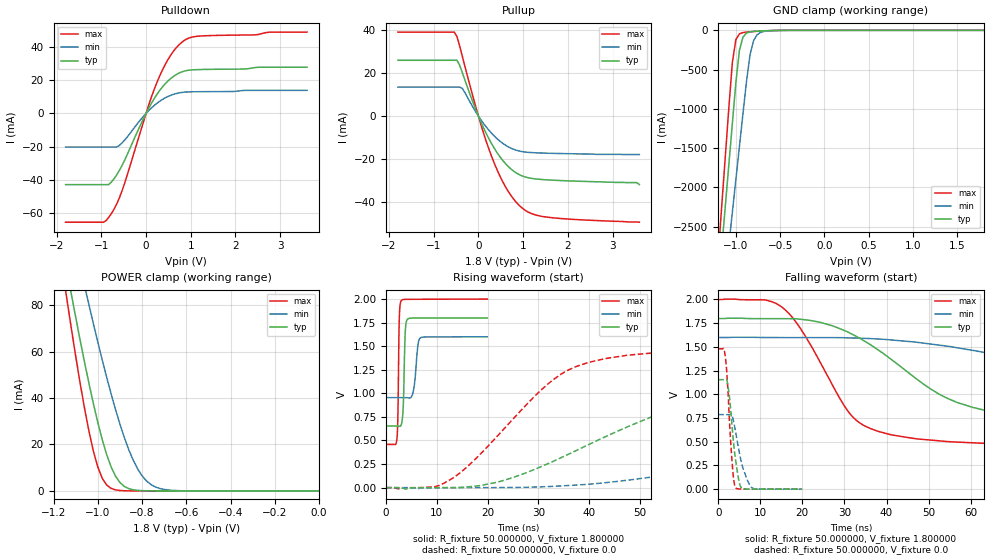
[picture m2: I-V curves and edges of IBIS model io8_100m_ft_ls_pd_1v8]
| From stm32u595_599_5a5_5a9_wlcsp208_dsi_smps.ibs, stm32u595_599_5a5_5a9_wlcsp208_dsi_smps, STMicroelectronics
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|   Model io8_100m_ft_ls_pd_1v8
[Model]  io8_100m_ft_ls_pd_1v8
Model_type I/O
Polarity   Non-Inverting
Enable   Active-Low
Vinl =   0.540000V
Vinh =   1.260000V
Vmeas =  0.900000V
Cref =   50.000000pF
Rref =   100.000000M
Vref =   0.0V
C_comp   3.148300pF   3.147400pF   3.196500pF
[Temperature Range]   25.000000   0.140000k   -40.000000
[Pullup Reference]   1.800000V   1.600000V   2.000000V
[Pulldown Reference]   0.0V   0.0V   0.0V
[POWER Clamp Reference]   1.800000V   1.600000V   2.000000V
[GND Clamp Reference]   0.0V   0.0V   0.0V
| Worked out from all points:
|   slope of the pulldown table from 0 to 0.27 V, typ, clamps not added: 21.7 ohm
|   slope of the pullup table from 0 to 0.27 V, typ, clamps not added: 22.6 ohm
|   GND clamp passes 1 mA (typ) near -0.51 V on its own axis
|   POWER clamp passes 1 mA (typ) near -0.86 V on its own axis
|   rising waveform, R_fixture 50.000000, V_fixture 1.800000: 20-80 % time 318ps typ, 631ps min, 230ps max; typ from 0.654 V to 1.8 V
|   rising waveform, R_fixture 50.000000, V_fixture 0.0: 20-80 % time 31.3ns typ, 66.8ns min, 16.5ns max; typ from 0 V to 1.15 V
|   falling waveform, R_fixture 50.000000, V_fixture 1.800000: 20-80 % time 24.6ns typ, 55.5ns min, 12.3ns max; typ from 1.8 V to 0.654 V
|   falling waveform, R_fixture 50.000000, V_fixture 0.0: 20-80 % time 1.6ns typ, 2.38ns min, 1.17ns max; typ from 1.15 V to 0 V
[Pulldown]
|Voltage   I(typ)   I(min)   I(max)
-1.8V     -42.74mA   -20.21mA   -65.25mA
-960mV    -42.74mA   -20.21mA   -65.25mA
-780mV    -41.3mA    -20.21mA   -60.25mA
-660mV    -37mA      -20.2mA    -54.5mA
-540mV    -31.39mA   -17.82mA   -46.65mA
0V        0A         0A         0A
240mV     11.28mA    6.002mA    18.38mA
480mV     19.17mA    10.02mA    31.83mA
780mV     24.67mA    12.5mA     42.21mA
960mV     25.9mA     12.9mA     45.21mA
1.14V     26.24mA    12.99mA    46.23mA
3.6V      27.67mA    13.81mA    48.75mA
[Pullup]
|Voltage   I(typ)   I(min)   I(max)
-1.8V     26.06mA    13.5mA     39.23mA
-540mV    26.06mA    13.5mA     39.23mA
-480mV    26.06mA    13.5mA     37.19mA
-360mV    20.34mA    12.93mA    27.94mA
0V        0A         0A         0A
300mV     -13.1mA    -8.158mA   -19.11mA
480mV     -18.98mA   -11.71mA   -27.97mA
660mV     -23.42mA   -14.29mA   -34.95mA
1.02V     -28.29mA   -16.75mA   -43.65mA
1.26V     -29.33mA   -17.15mA   -46.11mA
1.62V     -29.92mA   -17.41mA   -47.45mA
3.6V      -32mA      -18mA      -49.6mA
[GND_clamp]
|Voltage   I(typ)   I(min)   I(max)
-1.8V     -9.707A    -9.942A    -9.774A
-1.2V     -3.309A    -4.006A    -2.865A
-1.16V    -2.777A    -3.584A    -2.239A
-1.12V    -2.246A    -3.162A    -1.614A
-1.04V    -1.186A    -2.319A    -408.7mA
-1V       -663.9mA   -1.898A    -117.8mA
-960mV    -254mA     -1.478A    -45.15mA
-920mV    -86.04mA   -1.06A     -28.6mA
-840mV    -19.13mA   -308.9mA   -18.75mA
-800mV    -13.4mA    -130.8mA   -15.33mA
-720mV    -7.959mA   -25.38mA   -9.395mA
1.8V      45.71uA    33.33uA    56.11uA
[POWER_clamp]
|Voltage   I(typ)   I(min)   I(max)
-1.8V     470.8mA    433.7mA    554.6mA
-1.14V    95.25mA    122.7mA    82.82mA
-1.12V    84.97mA    114mA      70.27mA
-1.06V    55.51mA    88.42mA    35.67mA
-1.04V    46.34mA    80.15mA    25.76mA
-1V       29.51mA    64.13mA    10.3mA
-940mV    10.39mA    41.86mA    1.109mA
-900mV    3.624mA    28.77mA    182.8uA
-840mV    490.7uA    13.24mA    11.35uA
-800mV    116.8uA    6.532mA    1.77uA
-740mV    13.2uA     1.723mA    109.3nA
0V        0A         18.72nA    0A
[Ramp]
| variable   typ   min   max
dV/dt_r  0.69258/31.23580n   0.47167/66.68725n   0.88830/16.46503n
dV/dt_f  0.68752/24.55124n   0.38681/55.45968n   0.92452/12.26326n
R_load = 50.000000
[Rising Waveform]
R_fixture= 50.000000
V_fixture= 1.800000
V_fixture_min= 1.600000
V_fixture_max= 2.000000
|time   V(typ)   V(min)   V(max)
0s        653.5mV    954.4mV    458.4mV
2.202ns   653.4mV    954.4mV    531.4mV
2.362ns   653.1mV    954.4mV    755.2mV
2.643ns   650.8mV    954.4mV    1.796V
3.043ns   670mV      954.5mV    1.984V
3.443ns   892.3mV    954.4mV    1.994V
3.844ns   1.677V     954.2mV    1.996V
4.204ns   1.783V     953.1mV    1.996V
6.807ns   1.799V     1.589V     1.997V
19.94ns   1.799V     1.599V     1.999V
[Rising Waveform]
R_fixture= 50.000000
V_fixture= 0.0
V_fixture_min= 0.0
V_fixture_max= 0.0
|time   V(typ)   V(min)   V(max)
0s        2.158nV    142.4nV    1.475nV
9.61ns    -281.8uV   -154.3uV   10.23mV
13.61ns   914.2uV    -130.3uV   117mV
23.22ns   77.25mV    902.5uV    623mV
36.04ns   357.8mV    23.07mV    1.251V
54.45ns   794.3mV    128.7mV    1.437V
81.68ns   1.078V     359.9mV    1.475V
120.1ns   1.142V     609.8mV    1.48V
153ns     1.152V     713.5mV    1.48V
398.8ns   1.154V     786.2mV    1.48V
[Falling Waveform]
R_fixture= 50.000000
V_fixture= 1.800000
V_fixture_min= 1.600000
V_fixture_max= 2.000000
|time   V(typ)   V(min)   V(max)
0s        1.799V     1.599V     1.999V
15.22ns   1.798V     1.598V     1.918V
20.02ns   1.789V     1.598V     1.662V
32.03ns   1.629V     1.594V     758.4mV
37.64ns   1.479V     1.584V     614.7mV
47.25ns   1.158V     1.549V     529.9mV
63.26ns   832.8mV    1.441V     483.3mV
100.1ns   689.8mV    1.14V      461.4mV
176.2ns   655.9mV    987.3mV    458.4mV
398.8ns   653.5mV    954.4mV    458.4mV
[Falling Waveform]
R_fixture= 50.000000
V_fixture= 0.0
V_fixture_min= 0.0
V_fixture_max= 0.0
|time   V(typ)   V(min)   V(max)
0s        1.154V     786.2mV    1.48V
1.281ns   1.154V     786.2mV    1.485V
1.682ns   1.155V     786.2mV    1.399V
2.402ns   1.066V     786mV      970.3mV
3.363ns   631.9mV    766.9mV    250mV
3.764ns   438.3mV    691mV      74.59mV
4.164ns   299.8mV    596.6mV    14.88mV
5.285ns   30.89mV    328.5mV    1.27mV
7.888ns   345.5uV    19.66mV    100.4uV
19.94ns   2.158nV    142.4nV    1.475nV
